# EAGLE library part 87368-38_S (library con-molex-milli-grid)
RECEPTACAL
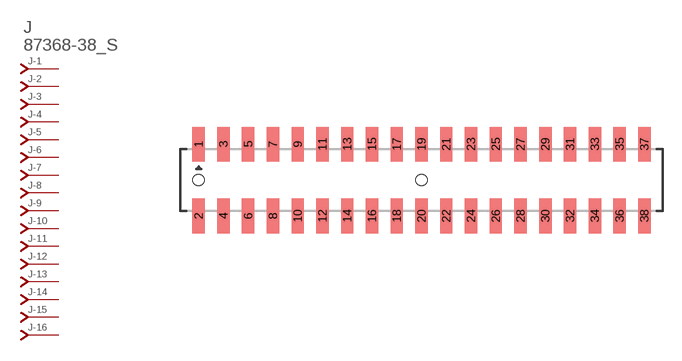
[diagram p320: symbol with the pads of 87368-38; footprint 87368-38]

Designator prefix J; gates -1=J-NV -2=J-N -3=J-N -4=J-N -5=J-N -6=J-N -7=J-N -8=J-N -9=J-N -10=J-N -11=J-N -12=J-N -13=J-N -14=J-N -15=J-N -16=J-N -17=J-N -18=J-N -19=J-N -20=J-N -21=J-N -22=J-N -23=J-N -24=J-N -25=J-N -26=J-N -27=J-N -28=J-N -29=J-N -30=J-N -31=J-N -32=J-N -33=J-N -34=J-N -35=J-N -36=J-N -37=J-N -38=J-N

## 87368-38_S  [87368-38]
1  -1:J  pas
2  -2:J  pas
3  -3:J  pas
4  -4:J  pas
5  -5:J  pas
6  -6:J  pas
7  -7:J  pas
8  -8:J  pas
9  -9:J  pas
10  -10:J  pas
11  -11:J  pas
12  -12:J  pas
13  -13:J  pas
14  -14:J  pas
15  -15:J  pas
16  -16:J  pas
17  -17:J  pas
18  -18:J  pas
19  -19:J  pas
20  -20:J  pas
21  -21:J  pas
22  -22:J  pas
23  -23:J  pas
24  -24:J  pas
25  -25:J  pas
26  -26:J  pas
27  -27:J  pas
28  -28:J  pas
29  -29:J  pas
30  -30:J  pas
31  -31:J  pas
32  -32:J  pas
33  -33:J  pas
34  -34:J  pas
35  -35:J  pas
36  -36:J  pas
37  -37:J  pas
38  -38:J  pas

## Footprint 87368-38 (pad centres in mm)
RECEPTACAL SMD Dual Row, Side Entry
smd 1 x 2.8: 1 -18,2.9; 2 -18,-2.9; 3 -16,2.9; 4 -16,-2.9; 5 -14,2.9; 6 -14,-2.9; 7 -12,2.9; 8 -12,-2.9; 9 -10,2.9; 10 -10,-2.9; 11 -8,2.9; 12 -8,-2.9; 13 -6,2.9; 14 -6,-2.9; 15 -4,2.9; 16 -4,-2.9; 17 -2,2.9; 18 -2,-2.9; 19 0,2.9; 20 0,-2.9; 21 2,2.9; 22 2,-2.9; 23 4,2.9; 24 4,-2.9; 25 6,2.9; 26 6,-2.9; 27 8,2.9; 28 8,-2.9; 29 10,2.9; 30 10,-2.9; 31 12,2.9; 32 12,-2.9; 33 14,2.9; 34 14,-2.9; 35 16,2.9; 36 16,-2.9; 37 18,2.9; 38 18,-2.9
hole 0.914 at -18,0
hole 0.914 at 0,0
